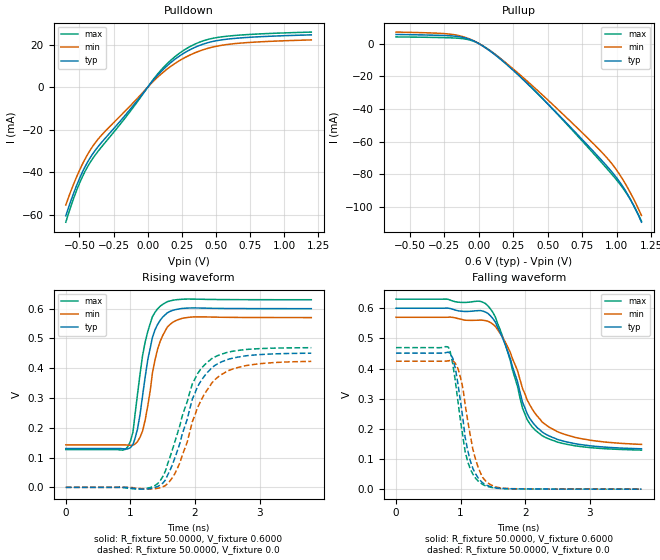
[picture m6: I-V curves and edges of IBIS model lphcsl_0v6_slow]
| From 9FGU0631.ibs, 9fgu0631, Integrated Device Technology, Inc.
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[Model]  lphcsl_0v6_slow
Model_type Output
Polarity   Non-Inverting
Enable   Active-High
Vmeas =  0.4000V
Cref =   2.0000pF
Rref =   0.0
Vref =   0.4000V
C_comp   1.1000pF   1.0000pF   1.2000pF
[Temperature Range]   25.0000   75.0000   0.0
[Voltage Range]   0.6000V   0.5700V   0.6300V
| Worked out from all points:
|   slope of the pulldown table from 0 to 0.09 V, typ, clamps not added: 13.2 ohm
|   slope of the pullup table from 0 to 0.09 V, typ, clamps not added: 17.6 ohm
|   rising waveform, R_fixture 50.0000, V_fixture 0.6000: 20-80 % time 212ps typ, 222ps min, 215ps max; typ from 0.13 V to 0.6 V
|   rising waveform, R_fixture 50.0000, V_fixture 0.0: 20-80 % time 428ps typ, 456ps min, 422ps max; typ from 0 V to 0.45 V
|   falling waveform, R_fixture 50.0000, V_fixture 0.6000: 20-80 % time 457ps typ, 529ps min, 424ps max; typ from 0.6 V to 0.134 V
|   falling waveform, R_fixture 50.0000, V_fixture 0.0: 20-80 % time 206ps typ, 223ps min, 200ps max; typ from 0.451 V to 0 V
[Pulldown]
|Voltage   I(typ)   I(min)   I(max)
-600mV    -60.47mA   -55.34mA   -63.45mA
-540mV    -49.36mA   -45.1mA    -51.8mA
-500mV    -42.97mA   -39.12mA   -45.21mA
-440mV    -35.14mA   -31.55mA   -37.31mA
-380mV    -29.3mA    -25.74mA   -31.48mA
-140mV    -11.3mA    -9.552mA   -12.37mA
60mV      4.726mA    3.957mA    5.199mA
220mV     14.11mA    12mA       15.38mA
360mV     19.15mA    16.55mA    20.68mA
500mV     21.85mA    19.24mA    23.3mA
740mV     23.48mA    21.06mA    24.82mA
1.2V      24.65mA    22.28mA    25.96mA
[Pullup]
|Voltage   I(typ)   I(min)   I(max)
-600mV    5.539mA    7.002mA    4.049mA
-160mV    4.38mA     5.132mA    3.309mA
-40mV     1.727mA    1.805mA    1.473mA
100mV     -5.748mA   -5.607mA   -5.36mA
240mV     -15.68mA   -14.9mA    -15.23mA
420mV     -30.15mA   -28.26mA   -30.01mA
740mV     -57.84mA   -53.76mA   -58.73mA
920mV     -74.2mA    -69.1mA    -75.68mA
1V        -82.24mA   -77.52mA   -83.58mA
1.06V     -89.61mA   -85.43mA   -90.31mA
1.12V     -98.68mA   -94.71mA   -98.6mA
1.18V     -109.4mA   -105.3mA   -108.8mA
[Ramp]
| variable   typ   min   max
dV/dt_r  0.2702/0.4640n   0.2537/0.4902n   0.2813/0.4561n
dV/dt_f  0.2796/0.4910n   0.2529/0.5599n   0.3002/0.4601n
R_load = 50.0000
[Rising Waveform]
R_fixture= 50.0000
V_fixture= 0.6000
V_fixture_min= 0.5700
V_fixture_max= 0.6300
|time   V(typ)   V(min)   V(max)
0s        130.4mV    142.8mV    126.9mV
960ps     129.1mV    141.9mV    136.3mV
1.04ns    143.8mV    141.5mV    186.1mV
1.11ns    195.9mV    153.7mV    312.8mV
1.23ns    372.8mV    227.7mV    489.6mV
1.34ns    502.8mV    382.8mV    572.4mV
1.5ns     571.7mV    509.7mV    614.4mV
1.65ns    593.9mV    553.3mV    627.9mV
1.92ns    602.2mV    571.3mV    632.2mV
3.8ns     600mV      570mV      630mV
[Rising Waveform]
R_fixture= 50.0000
V_fixture= 0.0
V_fixture_min= 0.0
V_fixture_max= 0.0
|time   V(typ)   V(min)   V(max)
0s        0V         0V         0V
1.15ns    -5.145mV   -3.883mV   -6.088mV
1.46ns    7.325mV    -1.168mV   21.55mV
1.69ns    99.8mV     46.9mV     154.3mV
1.88ns    228.9mV    152.3mV    287.7mV
1.96ns    297.2mV    221.2mV    348.3mV
2.19ns    385.7mV    327.8mV    419.7mV
2.38ns    418.1mV    374.5mV    444.8mV
2.65ns    436.8mV    401.6mV    459.1mV
3.8ns     450.4mV    422.9mV    468.9mV
[Falling Waveform]
R_fixture= 50.0000
V_fixture= 0.6000
V_fixture_min= 0.5700
V_fixture_max= 0.6300
|time   V(typ)   V(min)   V(max)
0s        600mV      570mV      630mV
1.38ns    587.9mV    559.2mV    616.2mV
1.54ns    553.5mV    539.5mV    569.9mV
1.69ns    479.7mV    488.5mV    480.8mV
1.88ns    357.8mV    393.9mV    341.9mV
1.96ns    287.4mV    333.2mV    267.5mV
2.15ns    212.4mV    252.3mV    197mV
2.34ns    179.8mV    210.2mV    168.9mV
2.65ns    156.4mV    179.2mV    148.6mV
3.8ns     134mV      148.5mV    129.6mV
[Falling Waveform]
R_fixture= 50.0000
V_fixture= 0.0
V_fixture_min= 0.0
V_fixture_max= 0.0
|time   V(typ)   V(min)   V(max)
0s        451.1mV    424.4mV    469.3mV
810ps     454.3mV    425.5mV    471.2mV
880ps     433.5mV    426mV      414.2mV
920ps     398.9mV    417.2mV    356.3mV
1ns       288.4mV    368.8mV    224.5mV
1.07ns    172.1mV    280.7mV    125.3mV
1.19ns    68.93mV    132.7mV    49.98mV
1.34ns    21.11mV    39.57mV    15.76mV
1.69ns    1.913mV    2.778mV    1.596mV
3.8ns     62.81uV    95.66uV    49.56uV
